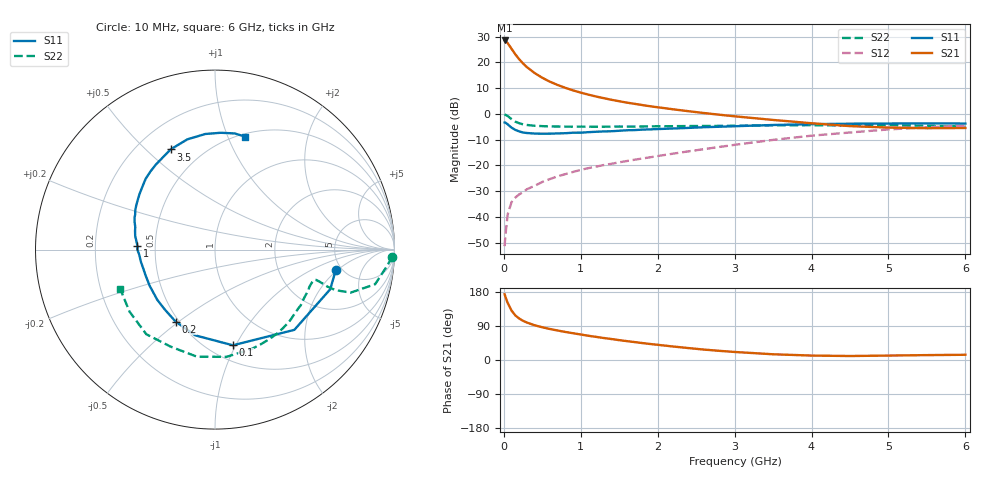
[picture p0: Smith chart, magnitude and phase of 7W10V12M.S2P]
! Infineon Technologies  Discrete & RF Semiconductors
! BFS17W
! Si NPN RF Bipolar Junction Transistor in SOT323
! VCE = 10 V  IC = 12 mA
! Common Emitter S-Parameters:  August  1999
# GHz  S  MA  R  50
!  f  S11  S21  S12  S22
! GHz  MAG  ANG  MAG  ANG  MAG  ANG  MAG  ANG
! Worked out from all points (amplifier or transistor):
!   36 points, 10 MHz to 6 GHz, reference 50 ohm
!   highest |S21| = 28.6 dB at 10 MHz (marker M1)
!   |S21| within 3 dB of that: start of sweep to 94.76 MHz
!   unconditionally stable (mu >= 1): 392.3 MHz to 2.081 GHz; 5.659 GHz to end of sweep
!   at 250 MHz: K = 0.83, MSG = 25.0 dB, |S12| = -30.4 dB
!   at 1.4 GHz: K = 1.16, MAG = 10.0 dB, |S12| = -19.4 dB
!   at 6 GHz: K = 1.03, MAG = -1.5 dB, |S12| = -4.5 dB
!   S11 on the Smith chart (normalised r, x): 10 MHz: 4.47, -1.89; 100 MHz: 0.64, -0.97; 200 MHz: 0.48, -0.49; 1 GHz: 0.40, +0.02; 3.5 GHz: 0.34, +0.60; 6 GHz: 0.53, +1.16
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0.01  0.6826 -9.5  26.78 173.6  0.0027 82.3  0.9889 -2.3
0.02  0.6789 -19.0  26.31 167.1  0.0043 85.9  0.9633 -5.4
0.05  0.6288 -45.3  23.79 150.4  0.0112 69.1  0.9127 -12.2
0.1  0.5424 -79.4  18.46 130.5  0.0194 62.0  0.793 -17.6
0.15  0.4903 -102.9  14.36 117.6  0.0238 57.4  0.7074 -18.6
0.2  0.4575 -118.6  11.55 109.4  0.0274 56.8  0.6587 -18.2
0.25  0.4355 -129.9  9.55 103.4  0.0302 57.1  0.6286 -17.5
0.3  0.4264 -138.9  8.123 98.8  0.0345 58.9  0.611 -17.1
0.4  0.4161 -151.2  6.236 91.7  0.0402 61.5  0.5892 -16.7
0.5  0.4125 -159.9  5.044 86.3  0.0478 63.4  0.58 -16.9
0.6  0.4139 -166.2  4.227 81.8  0.0544 65.6  0.573 -17.7
0.7  0.4189 -171.1  3.652 77.8  0.0615 66.6  0.5698 -18.8
0.8  0.4225 -175.9  3.215 74.0  0.0678 67.5  0.5676 -20.2
1  0.4329 177.1  2.594 67.3  0.082 69.1  0.5673 -23.2
1.1  0.4428 173.0  2.371 63.9  0.0886 69.4  0.566 -25.1
1.6  0.482 158.5  1.659 49.8  0.1219 71.5  0.5681 -35.3
2.2  0.5218 143.8  1.232 35.6  0.1693 73.8  0.5791 -49.4
2.8  0.5646 129.6  0.967 24.2  0.2284 73.3  0.5863 -64.8
3.5  0.6105 113.9  0.765 15.1  0.3136 69.3  0.601 -83.8
4.5  0.6464 94.8  0.58 10.5  0.4364 57.6  0.5945 -114.6
5.5  0.6563 80.4  0.528 12.9  0.5509 44.3  0.5884 -144.1
6  0.6514 74.9  0.534 13.8  0.5958 37.6  0.5715 -157.5
